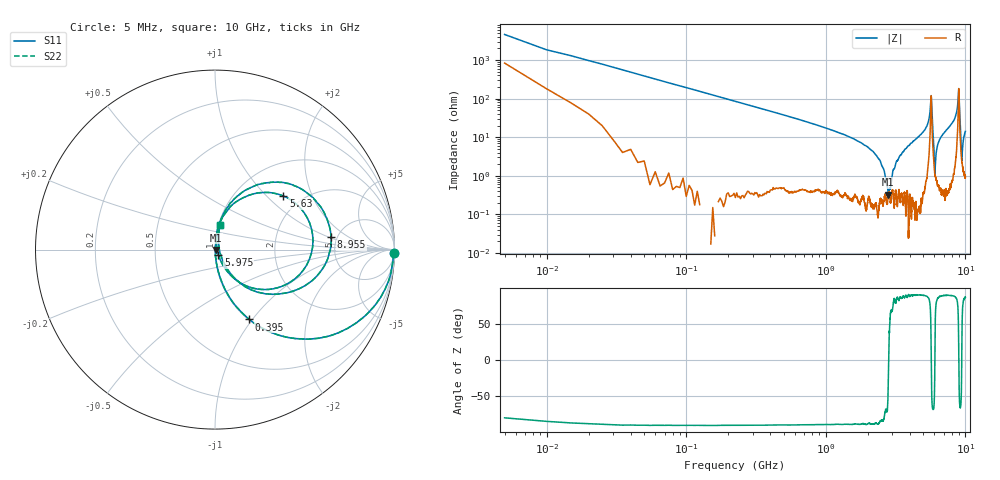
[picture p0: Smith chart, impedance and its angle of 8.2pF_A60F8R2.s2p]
! Amotech Co.,Ltd.
! http://www.amotech.co.kr/
! Part Number: A60F8R2
! These Parameters are Measured in Series Mode Connection
! Operation Temp=25[degC], DC Bias Voltage=0[V]
! Freq. Start=5[MHz] Stop=10[GHz], 2000[Steps]
! Date: Monday, July 20, 2020, 03:32:06
# GHZ S RI R 50.000000
!Freq.(Hz) S11(Real) S11(Imag) S21(Real) S21(Imag) S12(Real) S12(Imag) S22(Real) S22(Imag)
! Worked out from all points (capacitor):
!   2000 points, 5 MHz to 10 GHz, reference 50 ohm
!   read as one part in series: C = 8.24 pF near 55 MHz
!   lowest |Z| = 328 mohm at 2.805 GHz (marker M1)
!   series resonance near 2.82 GHz, so ESL is about 390 pH
!   S11 on the Smith chart (normalised r, x): 5 MHz: 18, -91; 395 MHz: 1.01, -0.97; 5.63 GHz: 1.62, +1.26; 5.975 GHz: 1.04, -0.06; 8.955 GHz: 4.44, +1.07; 10 GHz: 1.02, +0.28
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0.005  0.9956 -0.0211  0.00437 0.0211  0.00437 0.0211  0.9956 -0.0211
0.065  0.8975 -0.3024  0.1025 0.3024  0.1025 0.3024  0.8975 -0.3024
0.115  0.7389 -0.4387  0.2611 0.4387  0.2611 0.4387  0.7389 -0.4387
0.395  0.1909 -0.3892  0.8091 0.3892  0.8091 0.3892  0.1909 -0.3892
1.675  0.0092 -0.0803  0.9908 0.0803  0.9908 0.0803  0.0092 -0.0803
2.43  0.00247 -0.0256  0.9975 0.0256  0.9975 0.0256  0.00247 -0.0256
2.805  0.00295 -0.00141  0.9971 0.00141  0.9971 0.00141  0.00295 -0.00141
3.34  0.00526 0.0291  0.9947 -0.0291  0.9947 -0.0291  0.00526 0.0291
5.005  0.0226 0.1365  0.9774 -0.1365  0.9774 -0.1365  0.0226 0.1365
5.465  0.0925 0.2462  0.9075 -0.2462  0.9075 -0.2462  0.0925 0.2462
5.63  0.3808 0.2987  0.6192 -0.2987  0.6192 -0.2987  0.3808 0.2987
5.755  0.2762 -0.2226  0.7238 0.2226  0.7238 0.2226  0.2762 -0.2226
5.975  0.0188 -0.0292  0.9812 0.0292  0.9812 0.0292  0.0188 -0.0292
6.06  0.01 0.00719  0.99 -0.00719  0.99 -0.00719  0.01 0.00719
6.24  0.00952 0.0482  0.9905 -0.0482  0.9905 -0.0482  0.00952 0.0482
6.67  0.0145 0.0983  0.9855 -0.0983  0.9855 -0.0983  0.0145 0.0983
8.335  0.0906 0.2641  0.9094 -0.2641  0.9094 -0.2641  0.0906 0.2641
8.81  0.3708 0.375  0.6292 -0.375  0.6292 -0.375  0.3708 0.375
8.955  0.6461 0.0696  0.3539 -0.0696  0.3539 -0.0696  0.6461 0.0696
9.08  0.3193 -0.2491  0.6807 0.2491  0.6807 0.2491  0.3193 -0.2491
9.42  0.0235 0.00247  0.9765 -0.00247  0.9765 -0.00247  0.0235 0.00247
10  0.0286 0.1363  0.9714 -0.1363  0.9714 -0.1363  0.0286 0.1363
